TYPE STR_FCSP700_INPUT :
STRUCT
	Active_Exception_Status	:	USINT	;
	Flow_Reading			:	REAL	;
	Pressure_Reading		:	REAL	;
	Temperature_Reading		:	REAL	;
	Position_Readback		:	REAL	;
	Position_Setpoint		:	REAL	;
	WcState					:	BIT		;
	InputToggle				:	BIT		;
	State					:	UINT	;
	//AdsAddr				:	AMSADDR	;
END_STRUCT
END_TYPE
